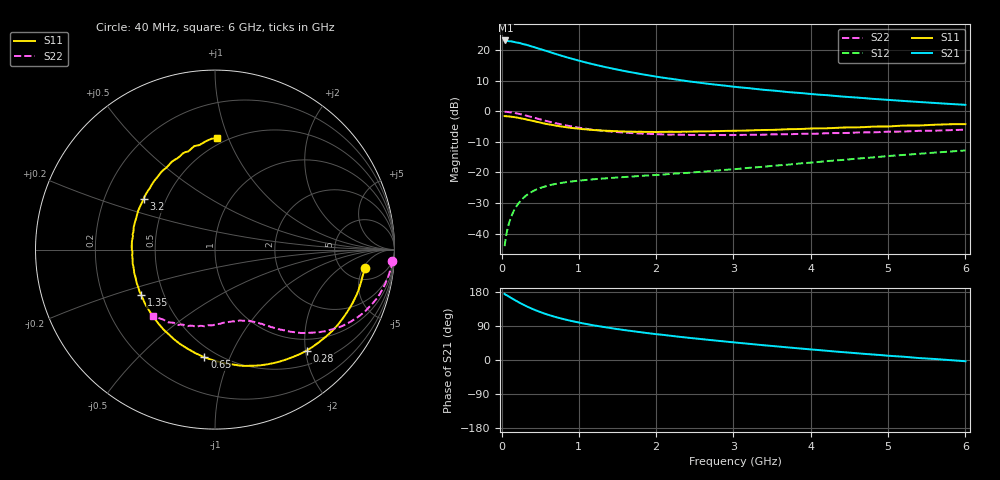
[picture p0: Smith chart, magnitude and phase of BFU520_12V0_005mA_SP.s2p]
! Filename:  P:\Prog\Test\Noise\ATS_data\Testdata_Net\03 Spar\BFU520_APG2013_37_A05_12p0V_005mA_SP_CM01_D.s2p
! Date/Time: Fri 26/Apr/2013 13:00:11
! BFU520_APG2013_37_A05_12p0V_1to20mA_SP_CM01_Bias4_R.s2p
! MDIF S-parameter v. bias file
! BFU520_APG2013_37_A05_12p0V_1to20mA_SP_CM01
! Date/time Tue Apr 23 18:22:57 2013
! VAR V_out= 12.0000
! VAR I_out= 4.9900
! VAR V_in= 0.8117
! VAR I_in= 0.0476
! Device data file deembeded for feedlines and parallel
! Original file: \03 Spar\BFU520_APG2013_37_A05_12p0V_005mA_SP_CM01_R.s2p
! Feed-files: PR047V01_250413_Feed1.s2p, PR047V01_250413_Feed2.s2p
! Parallel-file: PR047V01_250413_Par.s2p
# MHz S MA R 50
!  Freq-MHz  S11-mag  S11-arg  S21-mag  S21-arg  S12-mag  S12-arg  S22-mag  S22-arg
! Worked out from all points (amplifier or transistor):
!   98 points, 40 MHz to 6 GHz, reference 50 ohm
!   highest |S21| = 23.3 dB at 50 MHz (marker M1)
!   |S21| within 3 dB of that: start of sweep to 523.8 MHz
!   unconditionally stable (mu >= 1): 2.37 GHz to 4.422 GHz
!   at 300 MHz: K = 0.19, MSG = 25.0 dB, |S12| = -27.9 dB
!   at 1.6 GHz: K = 0.80, MSG = 17.3 dB, |S12| = -21.5 dB
!   at 6 GHz: K = 0.85, MSG = 7.5 dB, |S12| = -12.8 dB
!   S11 on the Smith chart (normalised r, x): 40 MHz: 7.66, -5.39; 280 MHz: 0.76, -2.02; 650 MHz: 0.43, -0.81; 1.35 GHz: 0.37, -0.24; 3.2 GHz: 0.37, +0.28; 6 GHz: 0.45, +0.91
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40  0.8399 -7.1  14.56 174.4  0.0062 82.9  0.989 -3.6
50  0.8373 -8.9  14.59 172.4  0.007669 82.6  0.9883 -4.7
70  0.8337 -12.3  14.36 170.7  0.01074 81.6  0.9826 -6.9
120  0.8223 -21.4  14.16 164.3  0.01811 77.5  0.9669 -11.6
180  0.8022 -31.6  13.62 157.3  0.02634 72.2  0.94 -17.0
240  0.7759 -41.6  13.18 150.4  0.03366 67.5  0.9062 -22.1
280  0.76 -47.8  12.71 146.3  0.03798 64.5  0.881 -25.2
340  0.7299 -56.9  12.18 140.2  0.04381 60.6  0.8419 -29.3
440  0.6846 -70.9  11.15 131.4  0.0518 55.0  0.7789 -35.2
550  0.6362 -84.8  10.09 122.8  0.05824 50.1  0.7133 -40.4
650  0.6031 -95.6  9.184 116.4  0.06313 46.8  0.6651 -44.3
850  0.55 -114.4  7.693 105.6  0.06983 42.4  0.5861 -49.9
1050  0.5133 -129.9  6.559 96.8  0.07457 39.8  0.5306 -54.3
1350  0.483 -148.6  5.322 86.2  0.08022 38.3  0.4766 -59.2
1600  0.4685 -161.7  4.578 78.6  0.0844 38.0  0.4493 -62.9
2050  0.4631 -179.9  3.639 67.2  0.09174 39.1  0.4223 -69.4
2450  0.4683 165.5  3.082 58.0  0.09938 40.5  0.4118 -75.6
3100  0.4846 146.5  2.473 44.7  0.1159 42.9  0.4128 -85.3
3200  0.4885 144.6  2.408 42.7  0.1193 43.2  0.4145 -86.6
4100  0.529 122.6  1.887 26.2  0.1488 43.5  0.4331 -101.4
5200  0.5881 101.4  1.488 8.6  0.1941 39.9  0.4684 -119.6
6000  0.6204 88.7  1.286 -3.3  0.2296 34.9  0.5029 -133.0
